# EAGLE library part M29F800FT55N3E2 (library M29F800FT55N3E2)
NOR Flash NOR Flash(Micron) , PARALLEL, 8M , TSOP 48PIN, 55ns, -40-+125C, TOP, Tray Source: Datasheet
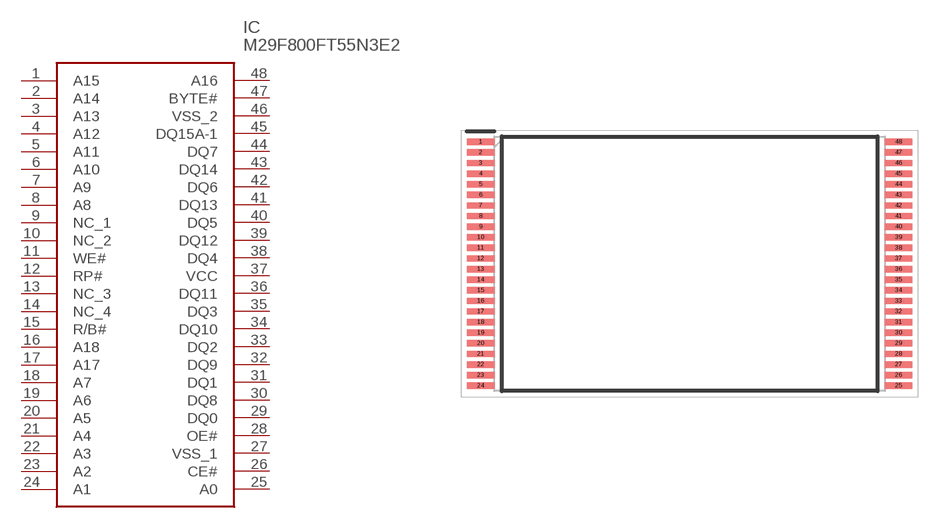
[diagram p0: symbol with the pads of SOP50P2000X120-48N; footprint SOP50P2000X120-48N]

Designator prefix IC

## M29F800FT55N3E2 (Description: NOR Flash NOR Flash(Micron) , PARALLEL, 8M , TSOP 48PIN, 55ns, -40-+125C, TOP, Tray; Height: 1.2mm; Manufacturer_Name: Alliance Memory; Manufacturer_Part_Number: M29F800FT55N3E2; Mouser_Part_Number: 913-M29F800FT55N3E2; Mouser_Price-Stock: https://www.mouser.co.uk/ProductDetail/Alliance-Memory/M29F800FT55N3E2?qs=vmHwEFxEFR9Aw9aI%2FlWRzQ%3D%3D)  [SOP50P2000X120-48N]
1  A15
2  A14
3  A13
4  A12
5  A11
6  A10
7  A9
8  A8
9  NC_1
10  NC_2
11  WE#
12  RP#
13  NC_3
14  NC_4
15  R/B#
16  A18
17  A17
18  A7
19  A6
20  A5
21  A4
22  A3
23  A2
24  A1
25  A0
26  CE#
27  VSS_1
28  OE#
29  DQ0
30  DQ8
31  DQ1
32  DQ9
33  DQ2
34  DQ10
35  DQ3
36  DQ11
37  VCC
38  DQ4
39  DQ12
40  DQ5
41  DQ13
42  DQ6
43  DQ14
44  DQ7
45  DQ15A-1
46  VSS_2
47  BYTE#
48  A16

## Footprint SOP50P2000X120-48N (pad centres in mm)
48-Lead TSOP &ndash; 12mm x 20mm
smd 1.3 x 0.3: 1 -9.85,5.75; 2 -9.85,5.25; 3 -9.85,4.75; 4 -9.85,4.25; 5 -9.85,3.75; 6 -9.85,3.25; 7 -9.85,2.75; 8 -9.85,2.25; 9 -9.85,1.75; 10 -9.85,1.25; 11 -9.85,0.75; 12 -9.85,0.25; 13 -9.85,-0.25; 14 -9.85,-0.75; 15 -9.85,-1.25; 16 -9.85,-1.75; 17 -9.85,-2.25; 18 -9.85,-2.75; 19 -9.85,-3.25; 20 -9.85,-3.75; 21 -9.85,-4.25; 22 -9.85,-4.75; 23 -9.85,-5.25; 24 -9.85,-5.75; 25 9.85,-5.75; 26 9.85,-5.25; 27 9.85,-4.75; 28 9.85,-4.25; 29 9.85,-3.75; 30 9.85,-3.25; 31 9.85,-2.75; 32 9.85,-2.25; 33 9.85,-1.75; 34 9.85,-1.25; 35 9.85,-0.75; 36 9.85,-0.25; 37 9.85,0.25; 38 9.85,0.75; 39 9.85,1.25; 40 9.85,1.75; 41 9.85,2.25; 42 9.85,2.75; 43 9.85,3.25; 44 9.85,3.75; 45 9.85,4.25; 46 9.85,4.75; 47 9.85,5.25; 48 9.85,5.75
